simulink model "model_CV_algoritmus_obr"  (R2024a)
settings: Solver=FixedStepAuto  StartTime=0.0  StopTime=inf  RelTol=1e-3  EnableMultiTasking=on
undefined symbols (not defined in the file): uint
libraries: visionsinks x2, deeplib x1, visionsources x1, visiontextngfix x1, dspstat3 x1

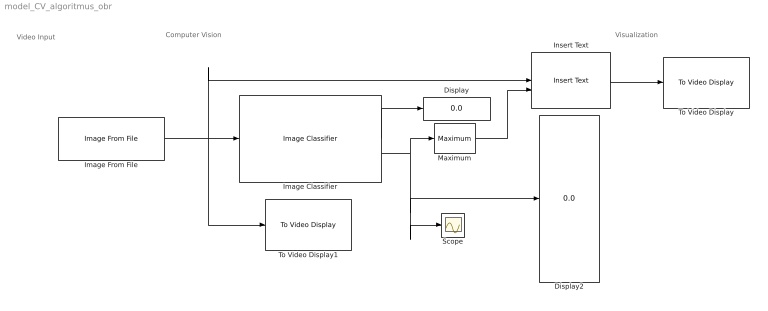
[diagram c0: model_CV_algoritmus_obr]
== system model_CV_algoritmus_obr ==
  note: Visualization
  note: Video Input
  note: Computer Vision
  Display : Display
  Display2 : Display
  Image Classifier : deeplib/Image Classifier  Network=Network from MAT-file  NetworkFunction=squeezenet  NetworkFilePath=trainedNetwork.mat  NetworkClassesVariable=classNames  MiniBatchSize=8  ResizeInput=on  Classification=on  Predictions=on  ForceInterpretedSim=off  PredictMode=All probabilities and labels  K=5
  Image From File : visionsources/Image From File  Tag=vipblks_nd  FileName=Hmozdinka.png  Ts=1/10  imagePorts=One multidimensional signal  OutPortLabels=R|G|B  ImageDataType=Inherit from input image  sdImageDataType=uint(8)  Signed=on  WordLength=16  FractionLengthMode=User-defined  FractionLength=15
  Insert Text : visiontextngfix/Insert Text  inputType=Obsolete  theText={'Hmozdinka','Hrebik','Matice','Matice kridlova','Podlozka','Prazdne','Sroub','Vrut'}  getTextLocFrom=Specify via dialog  textLoc=[1 1]  getTextColorFrom=Specify via dialog  textColor=[0 0 0]  getTextIntensityFrom=Specify via dialog  textIntensity=0  getTextOpacityFrom=Specify via dialog  textOpacity=1.0  dummyVar2=0  dummyVar3=0  dummyVar4=0  imagePorts=One multidimensional signal  isInputTransposed=off  fontFace=LucidaSansRegular  dummyVar1=0  blockFontSize=32  antiAliased=on
  Maximum : dspstat3/Maximum  operation=maximum  fcn=Index  indexBase=One  operateOver=Each row  Dimension=1  InputProcessing=Columns as channels (frame based)  reset=None  roiEnable=off  roiType=Rectangles  roiPortion=Entire ROI  roiOutput=Individual statistics for each ROI  roiFlag=off  roundingMode=Floor  overflowMode=off  accumDataTypeStr=Inherit: Same as product output  accumLastDataTypeStr=Inherit: Same as product output
  Scope : Scope
  To Video Display : visionsinks/To Video Display  windowSizeMode=Normal  openAtMdlStart=on  fullScreen=off  videoWindowX=1383  videoWindowY=404  saveWindowSize=off  videoWindowWidth=227  videoWindowHeight=227  inputColorFormat=RGB  inputType=Obsolete  imagePorts=One multidimensional signal  OutputDevice=On-screen video monitor  dataOrg=Column-major  isWindowOpen=off
  To Video Display1 : visionsinks/To Video Display  windowSizeMode=Normal  openAtMdlStart=on  fullScreen=off  videoWindowX=1150  videoWindowY=404  saveWindowSize=off  videoWindowWidth=227  videoWindowHeight=227  inputColorFormat=RGB  inputType=Obsolete  imagePorts=One multidimensional signal  OutputDevice=On-screen video monitor  dataOrg=Column-major  isWindowOpen=off
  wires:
  Image From File/1 -> Image Classifier/1, Insert Text/1, To Video Display1/1
  Image Classifier/1 -> Display/1
  Image Classifier/2 -> Maximum/1, Scope/1, Display2/1
  Insert Text/1 -> To Video Display/1
  Maximum/1 -> Insert Text/2
